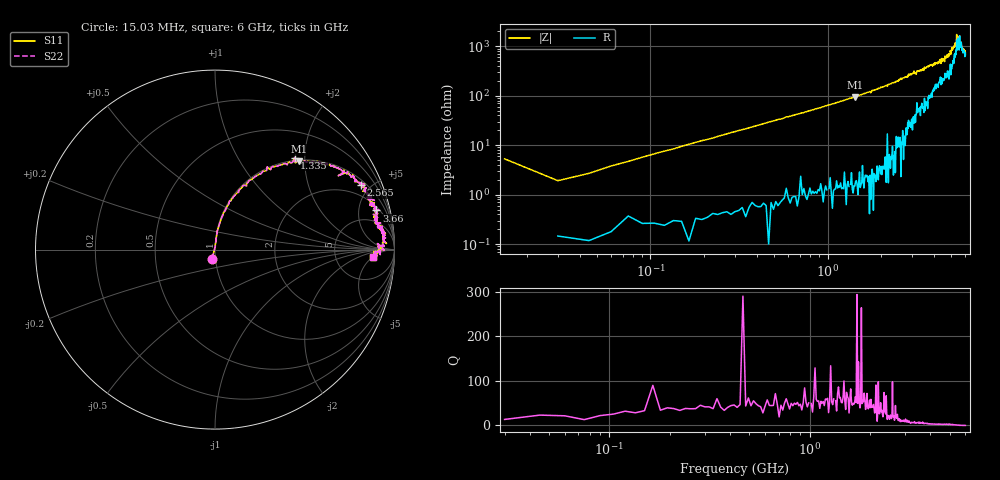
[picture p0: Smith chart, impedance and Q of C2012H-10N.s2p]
!	Network	Analyzer	HP8753E.07.74:	Oct	30	2002	Serial	No.	JP38451487
!	Hewlett-Packard
!	28	Aug	2009	9:41:42
!	Frequency	S11	S21	S12	S22
#	HZ	S	RI	R	50
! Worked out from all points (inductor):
!   400 points, 15.03 MHz to 6 GHz, reference 50 ohm
!   read as one part in series: L = 9.96 nH near 45.03 MHz
!   highest Q = 62.4 at 1.425 GHz (marker M1), where L = 10.4 nH
!   self-resonance near 5.561 GHz
!   S11 on the Smith chart (normalised r, x): 15.03 MHz: 0.96, -0.10; 1.335 GHz: 0.94, +1.79; 2.565 GHz: 1.29, +4.37; 3.66 GHz: 2.50, +7.55; 6 GHz: 14, -5
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1.502992e7  -0.0159 -0.0509  1.02 0.0509  1.02 0.0509  -0.0159 -0.0509
3.002985e7  0.00165 0.0191  0.998 -0.0191  0.998 -0.0191  0.00165 0.0191
1.050295e8  0.00714 0.0662  0.993 -0.0662  0.993 -0.0662  0.00714 0.0662
2.850286e8  0.035 0.173  0.965 -0.173  0.965 -0.173  0.035 0.173
1.020025e9  0.302 0.449  0.698 -0.449  0.698 -0.449  0.302 0.449
1.335023e9  0.444 0.513  0.556 -0.513  0.556 -0.513  0.444 0.513
1.425023e9  0.467 0.491  0.533 -0.491  0.533 -0.491  0.467 0.491
2.01002e9  0.68 0.454  0.32 -0.454  0.32 -0.454  0.68 0.454
2.565017e9  0.812 0.359  0.188 -0.359  0.188 -0.359  0.812 0.359
3.015015e9  0.872 0.3  0.128 -0.3  0.128 -0.3  0.872 0.3
3.660012e9  0.899 0.218  0.101 -0.218  0.101 -0.218  0.899 0.218
4.00501e9  0.906 0.179  0.0937 -0.179  0.0937 -0.179  0.906 0.179
5.010005e9  0.94 0.1  0.0603 -0.1  0.0603 -0.1  0.94 0.1
5.325003e9  0.936 0.0558  0.0637 -0.0558  0.0637 -0.0558  0.936 0.0558
5.355003e9  0.956 0.0336  0.0439 -0.0336  0.0439 -0.0336  0.956 0.0336
5.385003e9  0.941 0.0533  0.0588 -0.0533  0.0588 -0.0533  0.941 0.0533
5.520002e9  0.933 0.0152  0.0675 -0.0152  0.0675 -0.0152  0.933 0.0152
5.535002e9  0.905 0.0335  0.0948 -0.0335  0.0948 -0.0335  0.905 0.0335
5.565002e9  0.942 -0.00311  0.0577 0.00311  0.0577 0.00311  0.942 -0.00311
5.595002e9  0.908 0.019  0.0919 -0.019  0.0919 -0.019  0.908 0.019
5.685002e9  0.924 -0.00662  0.0762 0.00662  0.0762 0.00662  0.924 -0.00662
6e9  0.883 -0.0388  0.117 0.0388  0.117 0.0388  0.883 -0.0388
